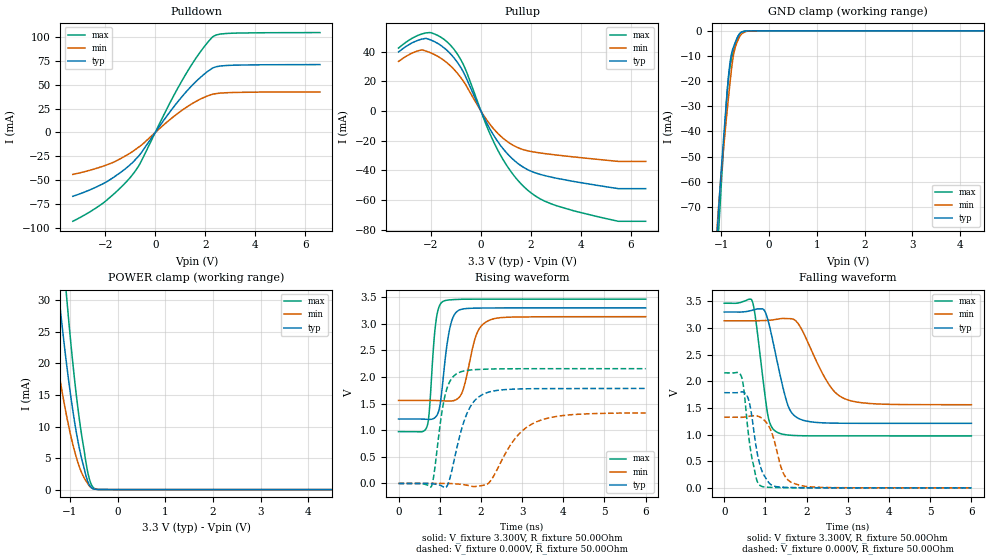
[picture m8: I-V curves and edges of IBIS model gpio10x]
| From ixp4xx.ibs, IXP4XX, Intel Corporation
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[Model]   gpio10x
Model_type   I/O
Vinl = 800.000mV
Vinh = 2.000V
Vmeas = 1.500V
Cref = 0.000F
|   typ   min   max
C_comp   3.000pF   2.700pF   3.300pF
[Voltage Range]   3.300V   3.135V   3.465V
[Temperature Range]   25.0   110.0   -40.0
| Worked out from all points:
|   slope of the pulldown table from 0 to 0.495 V, typ, clamps not added: 27 ohm
|   slope of the pullup table from 0 to 0.495 V, typ, clamps not added: 31.1 ohm
|   GND clamp passes 1 mA (typ) near -0.61 V on its own axis
|   POWER clamp passes 1 mA (typ) near -0.61 V on its own axis
|   falling waveform, V_fixture 3.300V, R_fixture 50.00Ohm: 20-80 % time 368ps typ, 624ps min, 240ps max; typ from 3.3 V to 1.21 V
|   rising waveform, V_fixture 3.300V, R_fixture 50.00Ohm: 20-80 % time 201ps typ, 292ps min, 137ps max; typ from 1.21 V to 3.3 V
|   rising waveform, V_fixture 0.000V, R_fixture 50.00Ohm: 20-80 % time 406ps typ, 726ps min, 248ps max; typ from 0 V to 1.79 V
|   falling waveform, V_fixture 0.000V, R_fixture 50.00Ohm: 20-80 % time 244ps typ, 301ps min, 215ps max; typ from 1.79 V to 0 V
[Pulldown]
|   Voltage   I(typ)   I(min)   I(max)
-3.3V     -66.86mA   -43.92mA   -93.01mA
-2.045V   -53.05mA   -34.89mA   -73.09mA
-1.33V    -40.71mA   -26.53mA   -56.36mA
-860mV    -30.17mA   -19.06mA   -42.52mA
-575mV    -21.75mA   -13.68mA   -30.9mA
510mV     18.88mA    11.8mA     27.08mA
1.11V     38.74mA    23.95mA    56.02mA
1.73V     55.83mA    33.94mA    81.64mA
2.3V      67.48mA    40.04mA    100.1mA
2.6V      69.58mA    41.22mA    103mA
3.115V    70.46mA    41.89mA    104mA
6.595V    71.12mA    42.53mA    104.7mA
[GND Clamp]
|   Voltage   I(typ)   I(min)   I(max)
-3.3V     -1.979A    -1.804A    -2.12A
-1.12V    -91.47mA   -86.95mA   -103.4mA
-1.08V    -77.94mA   -75.39mA   -87.8mA
-1.055V   -69.95mA   -68.92mA   -78.62mA
-995mV    -53.14mA   -54.78mA   -58.8mA
-895mV    -27.97mA   -34.71mA   -28.4mA
-845mV    -16.91mA   -25.39mA   -17.6mA
-790mV    -9.296mA   -15.53mA   -11.43mA
-740mV    -6.081mA   -8.954mA   -7.885mA
-670mV    -2.681mA   -4.492mA   -3.297mA
-570mV    -429.5uA   -1.119mA   -393.9uA
6.595V    0A         0A         0A
[Pullup]
|   Voltage   I(typ)   I(min)   I(max)
-3.3V     39.74mA    33.38mA    42.38mA
-2.585V   47.18mA    40.13mA    50.42mA
-2.2V     48.87mA    40.33mA    52.52mA
-1.745V   45.63mA    36.95mA    50.98mA
-1.255V   39.1mA     30.93mA    44.91mA
-700mV    26.15mA    20.02mA    31.14mA
190mV     -6.709mA   -4.987mA   -8.435mA
700mV     -21.19mA   -15.44mA   -27.12mA
1.4V      -34.21mA   -24.01mA   -45.08mA
2.11V     -41.2mA    -27.51mA   -56.35mA
4.715V    -50.16mA   -32.59mA   -71.23mA
6.595V    -52.21mA   -33.88mA   -74.18mA
[POWER Clamp]
|   Voltage   I(typ)   I(min)   I(max)
-3.3V     262.4mA    183.1mA    340.6mA
-1.465V   49.34mA    30.78mA    71.28mA
-1.24V    31.26mA    18.92mA    46.56mA
-1.215V   29.44mA    17.75mA    44.04mA
-1.07V    19.79mA    11.63mA    30.48mA
-930mV    12.02mA    6.853mA    19.28mA
-800mV    6.404mA    3.543mA    10.95mA
-630mV    1.332mA    997.1uA    2.826mA
-565mV    412.5uA    348.1uA    1.013mA
-515mV    136.2uA    138.7uA    344.2uA
-395mV    8.153uA    13.15uA    14.63uA
6.595V    0A         0A         0A
[Ramp]
R_load = 50.00Ohm
|   typ   min   max
dV/dt_r   1.071V/405.598ps 795.310mV/725.710ps   1.294V/248.145ps
dV/dt_f   1.254V/367.539ps 945.049mV/623.047ps   1.494V/239.282ps
[Falling Waveform]
V_fixture = 3.300V
V_fixture_min = 3.135V
V_fixture_max = 3.465V
R_fixture = 50.00Ohm
|   Time   V(typ)   V(min)   V(max)
0s        3.3V       3.135V     3.465V
680ps     3.333V     3.134V     3.505V
950ps     3.351V     3.139V     1.982V
1.06ns    3.153V     3.143V     1.359V
1.28ns    2.39V      3.164V     1.045V
1.58ns    1.485V     3.175V     989.2mV
1.9ns     1.272V     2.945V     978mV
2.49ns    1.218V     2.004V     975mV
2.92ns    1.212V     1.674V     975.2mV
6ns       1.211V     1.56V      974.6mV
[Rising Waveform]
V_fixture = 3.300V
V_fixture_min = 3.135V
V_fixture_max = 3.465V
R_fixture = 50.00Ohm
|   Time   V(typ)   V(min)   V(max)
0s        1.211V     1.56V      974.6mV
690ps     1.206V     1.561V     1.065V
750ps     1.204V     1.561V     1.383V
900ps     1.249V     1.56V      2.993V
1.08ns    1.944V     1.553V     3.422V
1.26ns    2.967V     1.549V     3.452V
1.49ns    3.265V     1.636V     3.461V
1.9ns     3.296V     2.817V     3.464V
2.2ns     3.299V     3.066V     3.465V
6ns       3.3V       3.135V     3.465V
[Rising Waveform]
V_fixture = 0.000V
V_fixture_min = 0.000V
V_fixture_max = 0.000V
R_fixture = 50.00Ohm
|   Time   V(typ)   V(min)   V(max)
0s        46.68nV    388.3nV    27.08nV
800ps     -5.139mV   213.9uV    -53.38mV
1.13ns    -83.1mV    610.2uV    1.657V
1.24ns    79.63mV    -926.3uV   1.909V
1.46ns    812.5mV    -12.36mV   2.082V
1.75ns    1.452V     -48.98mV   2.133V
2.19ns    1.717V     9.152mV    2.15V
2.83ns    1.774V     843.9mV    2.156V
3.33ns    1.782V     1.152V     2.157V
6ns       1.786V     1.326V     2.157V
[Falling Waveform]
V_fixture = 0.000V
V_fixture_min = 0.000V
V_fixture_max = 0.000V
R_fixture = 50.00Ohm
|   Time   V(typ)   V(min)   V(max)
0s        1.786V     1.326V     2.157V
420ps     1.801V     1.324V     2.083V
570ps     1.701V     1.338V     1.127V
660ps     1.395V     1.35V      613.1mV
790ps     698.2mV    1.349V     146.9mV
900ps     350mV      1.315V     31.33mV
1.14ns    57.2mV     1.062V     8.271mV
1.45ns    11.41mV    252mV      3.269mV
1.67ns    6.089mV    88.26mV    1.236mV
6ns       46.68nV    388.3nV    27.08nV
